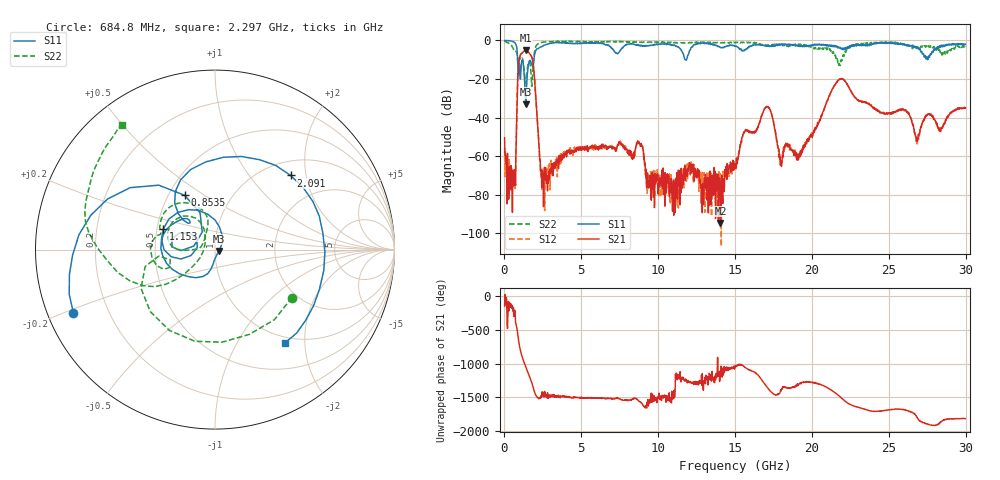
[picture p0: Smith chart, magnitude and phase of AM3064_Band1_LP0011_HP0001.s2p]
# Hz S DB R 50.0
!freq dBS11 angS11 dBS21 angS21 dBS12 angS12 dBS22 angS22
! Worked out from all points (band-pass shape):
!   1600 points, 10 MHz to 29.98 GHz, reference 50 ohm
!   highest |S21| = -5.23 dB at 1.378 GHz (marker M1); lowest = -94.6 dB at 14.05 GHz (marker M2)
!   |S21| within 3 dB of the highest: 1.013 GHz to 1.754 GHz (740.7 MHz wide, 53.5 % of centre)
!   lowest |S11| = -33.1 dB at 1.397 GHz (marker M3), VSWR 1.05, Z = 52.1 - j0.795 ohm
!   |S11| at or under -10 dB: 857.3 MHz to 1.914 GHz (1.057 GHz wide, 76.3 % of centre); 11.76 GHz to 11.84 GHz (83.91 MHz wide, 0.711 % of centre); 27.52448 GHz to 27.5319 GHz (7.425 MHz wide, 0.027 % of centre)
!   |S22| runs from -23.9 to -0.3 dB; largest |S21 - S12| = 0.0086
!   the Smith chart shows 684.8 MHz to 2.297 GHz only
!   S11 on the Smith chart (normalised r, x): 684.8 MHz: 0.08, -0.21; 853.5 MHz: 0.60, +0.41; 1.153 GHz: 0.54, +0.14; 2.091 GHz: 1.29, +1.63; 2.297 GHz: 0.90, -1.62
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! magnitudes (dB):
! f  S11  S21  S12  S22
! 10 MHz  0.0  -50.4  -55.6  -0.3
! 366.1 MHz  -0.2  -65.4  -72.6  -1.9
! 684.8 MHz  -1.3  -67.7  -76.8  -5.9
! 853.5 MHz  -9.2  -22.5  -22.4  -10.0
! 1.153 GHz  -10.2  -6.5  -6.5  -9.2
! 1.378 GHz  -30.7  -5.2  -5.2  -22.4
! 1.397 GHz  -33.1  -5.3  -5.2  -22.1
! 2.091 GHz  -4.6  -35.7  -35.7  -2.4
! 2.297 GHz  -3.7  -61.6  -62.2  -1.3
! 2.653 GHz  -2.3  -69.9  -66.0  -0.8
! 5.015 GHz  -1.5  -55.9  -55.3  -0.8
! 8.763 GHz  -2.8  -52.7  -53.1  -1.0
! 10 GHz  -2.0  -79.6  -71.0  -0.9
! 14.05 GHz  -3.6  -94.6  -72.9  -1.2
! 15 GHz  -2.9  -65.6  -64.6  -1.3
! 17.05 GHz  -2.8  -34.2  -34.2  -2.6
! 17.97 GHz  -2.5  -64.4  -62.7  -2.1
! 19.99 GHz  -2.8  -49.0  -48.5  -3.3
! 21.85 GHz  -3.6  -20.0  -19.9  -12.4
! 25 GHz  -1.1  -37.9  -37.6  -1.1
! 26.85 GHz  -4.3  -51.9  -53.7  -3.2
! 29.98 GHz  -1.9  -35.0  -35.0  -3.3
